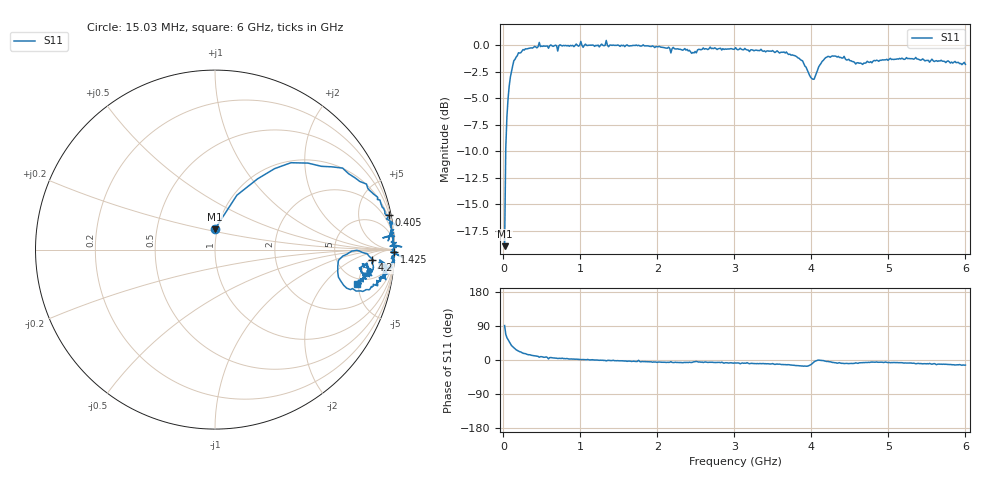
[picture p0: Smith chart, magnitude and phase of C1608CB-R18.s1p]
!	Network	Analyzer	HP8753E.07.74:	Oct	30	2002	Serial	No.	JP38451487
!	Hewlett-Packard
!	7	Sep	2009	10:03:13
!	Frequency	S11
#	HZ	S	RI	R	50
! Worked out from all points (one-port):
!   400 points, 15.03 MHz to 6 GHz, reference 50 ohm
!   lowest |S11| = -18.9 dB at 15.03 MHz (marker M1), VSWR 1.25, Z = 48.6 + j11.1 ohm
!   |S11| at or under -10 dB: start of sweep to 29.57 MHz
!   S11 on the Smith chart (normalised r, x): 15.03 MHz: 0.97, +0.22; 405 MHz: 1, +10; 1.425 GHz: open; 4.2 GHz: 12, -6; 6 GHz: 4.26, -4.71
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1.502992e7  -0.00146 0.113
3.002985e7  0.122 0.303
6.00297e7  0.332 0.451
9.002955e7  0.518 0.482
1.350293e8  0.711 0.454
1.95029e8  0.844 0.365
4.05028e8  0.967 0.191
5.550272e8  0.979 0.141
5.850271e8  0.965 0.0488
6.150269e8  0.995 0.113
7.050265e8  0.935 0.0655
7.650262e8  0.987 0.0816
1.245024e9  0.98 -0.0148
1.335023e9  1.05 -0.0452
1.425023e9  1 -0.0129
1.515022e9  0.985 -0.0367
2.265019e9  0.954 -0.106
2.505017e9  0.917 -0.058
3.015015e9  0.963 -0.134
3.765011e9  0.87 -0.208
3.93001e9  0.755 -0.223
4.02001e9  0.684 -0.0912
4.09501e9  0.79 -0.00433
4.200009e9  0.875 -0.0586
4.515007e9  0.833 -0.131
4.845006e9  0.845 -0.0754
5.265004e9  0.856 -0.123
6e9  0.789 -0.189
